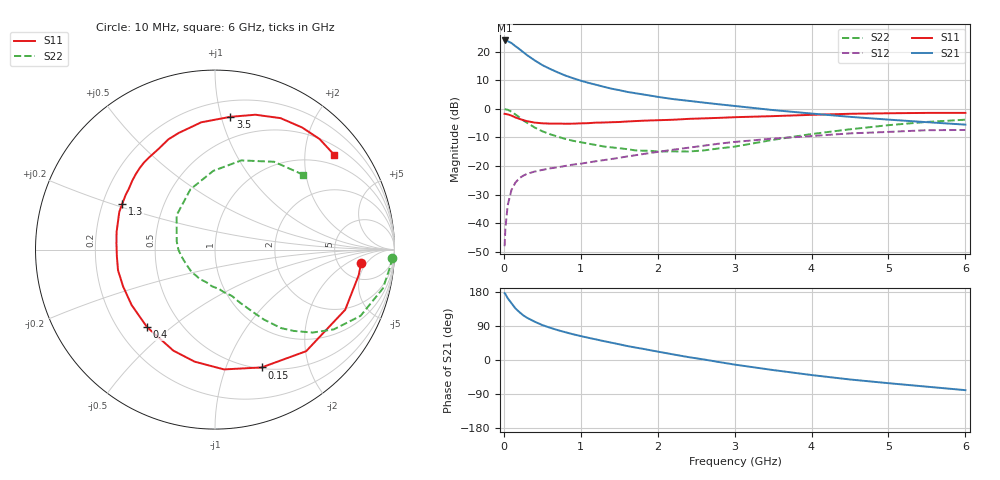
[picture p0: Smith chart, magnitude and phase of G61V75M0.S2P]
! SIEMENS Small Signal Semiconductors
! BFG193
! Si NPN RF Bipolar Junction Transistor in SOT223
! VCE = 1.75 V  IC = 5 mA
! Common Emitter S-Parameters:  August  1996
# GHz  S  MA  R  50
!  f  S11  S21  S12  S22
! GHz  MAG  ANG  MAG  ANG  MAG  ANG  MAG  ANG
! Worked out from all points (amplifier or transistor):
!   36 points, 10 MHz to 6 GHz, reference 50 ohm
!   highest |S21| = 23.9 dB at 10 MHz (marker M1)
!   |S21| within 3 dB of that: start of sweep to 201.7 MHz
!   unconditionally stable (mu >= 1): 1.085 GHz to 2.735 GHz
!   at 250 MHz: K = 0.34, MSG = 21.6 dB, |S12| = -23.4 dB
!   at 1.4 GHz: K = 1.09, MAG = 10.4 dB, |S12| = -17.5 dB
!   at 6 GHz: K = 0.93, MSG = 0.9 dB, |S12| = -7.4 dB
!   S11 on the Smith chart (normalised r, x): 10 MHz: 8.23, -3.75; 150 MHz: 0.51, -1.34; 400 MHz: 0.32, -0.41; 1.3 GHz: 0.28, +0.22; 3.5 GHz: 0.32, +1.07; 6 GHz: 0.71, +2.70
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0.01  0.8175 -5.3  15.59 176.5  0.004 91.3  0.9889 -2.7
0.02  0.8132 -10.1  15.55 174.1  0.0081 85.5  0.9815 -5.3
0.05  0.7991 -24.8  15.14 163.0  0.0207 76.5  0.9603 -13.0
0.1  0.7604 -48.1  14.03 149.7  0.0386 66.8  0.891 -24.5
0.15  0.7061 -68.4  12.41 136.3  0.0514 56.8  0.7969 -33.9
0.2  0.6694 -85.7  11.09 126.8  0.061 51.3  0.7133 -40.4
0.25  0.6346 -100.3  9.794 118.2  0.0678 46.3  0.631 -45.9
0.3  0.6089 -112.4  8.684 111.6  0.0731 43.1  0.5717 -49.9
0.4  0.5743 -131.3  7.012 101.2  0.0802 39.0  0.4724 -55.2
0.5  0.5579 -146.4  5.793 92.2  0.0857 36.1  0.4053 -58.8
0.6  0.5517 -158.1  4.974 85.2  0.0912 35.6  0.3604 -61.8
0.7  0.5525 -168.0  4.327 78.9  0.0952 35.2  0.3266 -64.8
0.9  0.5501 176.5  3.416 67.9  0.1061 35.1  0.2763 -69.7
1.1  0.5618 164.5  2.835 58.6  0.1158 35.3  0.2464 -77.1
1.3  0.5765 153.6  2.422 49.8  0.1273 35.3  0.2197 -84.3
1.6  0.6 140.2  1.978 37.1  0.1471 34.0  0.1978 -99.2
2.2  0.6438 119.0  1.478 14.8  0.1932 28.1  0.1807 -136.3
2.8  0.6948 101.2  1.196 -5.5  0.2466 18.6  0.2036 -179.5
3.5  0.7447 83.4  0.95 -26.5  0.3018 3.4  0.2872 138.1
4.5  0.8184 63.5  0.724 -51.4  0.3721 -16.8  0.4386 91.3
5.5  0.8479 46.6  0.584 -70.4  0.423 -41.4  0.5897 56.1
6  0.8485 38.5  0.529 -79.6  0.4269 -55.3  0.6453 40.2
